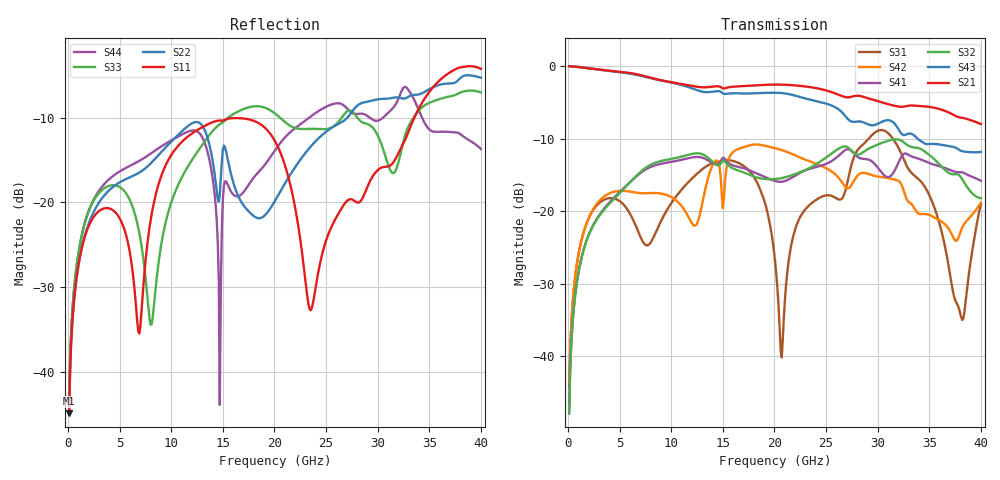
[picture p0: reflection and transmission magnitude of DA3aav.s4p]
! ADC12DJ2700AAV, ADC12DJ3200AAV, ADC08DJ3200AAV
! 144 pin AAV package
! Texas Instruments 4/21/2021
! Single-ended  S-parameters
! PORT#  PORT_NAME  NET_NAME
! PORT1:  DAxN.DIEBUMP DAxN
! PORT2:  DAxN.BGA  DAxN
! PORT3:  DAxP.DIEBUMP DAxP
! PORT4:  DAxP.BGA  DAxP
! Touchstone Ver. 1.0
! Number of ports is 4
# Hz	S	MA	R	50.000000
! SCATTERING PARAMETERS  :
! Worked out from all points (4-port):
!   400 points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, 100 MHz to 40 GHz, reference 50 ohm
!   strongest paths, dB at 100 MHz, 10.1 GHz, 20.1 GHz, 30.1 GHz, 40 GHz:
!     S21: 0.0, -2.2, -2.6, -4.9, -8.0
!     S43: 0.0, -2.3, -3.7, -7.9, -11.8
!     S32: -47.9, -12.8, -15.6, -10.8, -18.2
!     S41: -47.9, -13.2, -15.9, -14.2, -15.8
!     S42: -45.4, -18.1, -11.3, -15.2, -18.8
!     S31: -45.3, -18.7, -27.5, -8.9, -19.0
!   lowest |S11| = -44.9 dB at 100 MHz (marker M1), VSWR 1.01, Z = 50.2 + j0.528 ohm
!   |S11| at or under -10 dB: start of sweep to 33.54 GHz
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1e8  0.005699 67.3  0.9976 -1.7  0.005403 84.8  0.004048 -95.9
     0.9976 -1.7  0.005683 67.1  0.004048 -95.8  0.005399 85.3
     0.005403 84.8  0.004048 -95.8  0.006337 70.7  0.9977 -1.6
     0.004048 -95.9  0.005399 85.3  0.9977 -1.6  0.006312 70.8
8e9  0.07876 67.9  0.8301 -116.8  0.06078 178.9  0.2018 116.4
     0.8301 -116.8  0.1701 -36.4  0.2088 124.0  0.1332 -2.1
     0.06078 178.9  0.2088 124.0  0.01896 -174.0  0.8247 -114.2
     0.2018 116.4  0.1332 -2.1  0.8247 -114.2  0.1945 -20.8
1.35e10  0.2889 -23.0  0.7151 175.9  0.206 50.7  0.2251 16.2
         0.7151 175.9  0.2422 -153.0  0.2353 21.8  0.1631 128.5
         0.206 50.7  0.2353 21.8  0.2416 12.0  0.6606 178.6
         0.2251 16.2  0.1631 128.5  0.6606 178.6  0.2001 -165.5
1.47e10  0.3049 -40.6  0.7219 159.7  0.219 33.1  0.215 3.2
         0.7219 159.7  0.1109 -138.9  0.209 8.7  0.197 53.0
         0.219 33.1  0.209 8.7  0.2899 -6.2  0.6697 163.5
         0.215 3.2  0.197 53.0  0.6697 163.5  0.006372 67.4
1.52e10  0.3085 -46.8  0.7027 154.8  0.224 26.7  0.2281 -10.1
         0.7027 154.8  0.2125 -167.2  0.2196 -2.3  0.1577 86.1
         0.224 26.7  0.2196 -2.3  0.3058 -12.9  0.642 158.2
         0.2281 -10.1  0.1577 86.1  0.642 158.2  0.1332 177.2
2.07e10  0.1885 -146.4  0.7446 79.9  0.009826 20.4  0.1595 -76.7
         0.7446 79.9  0.1201 51.0  0.169 -59.1  0.2637 -0.9
         0.009826 20.4  0.169 -59.1  0.3106 -95.9  0.6512 87.6
         0.1595 -76.7  0.2637 -0.9  0.6512 87.6  0.2301 18.4
4e10  0.6163 -102.1  0.3984 164.7  0.1123 101.0  0.1618 -26.7
      0.3984 164.7  0.546 -109.0  0.1229 9.0  0.1143 31.3
      0.1123 101.0  0.1229 9.0  0.4468 -83.0  0.256 -132.9
      0.1618 -26.7  0.1143 31.3  0.256 -132.9  0.2069 -93.0
